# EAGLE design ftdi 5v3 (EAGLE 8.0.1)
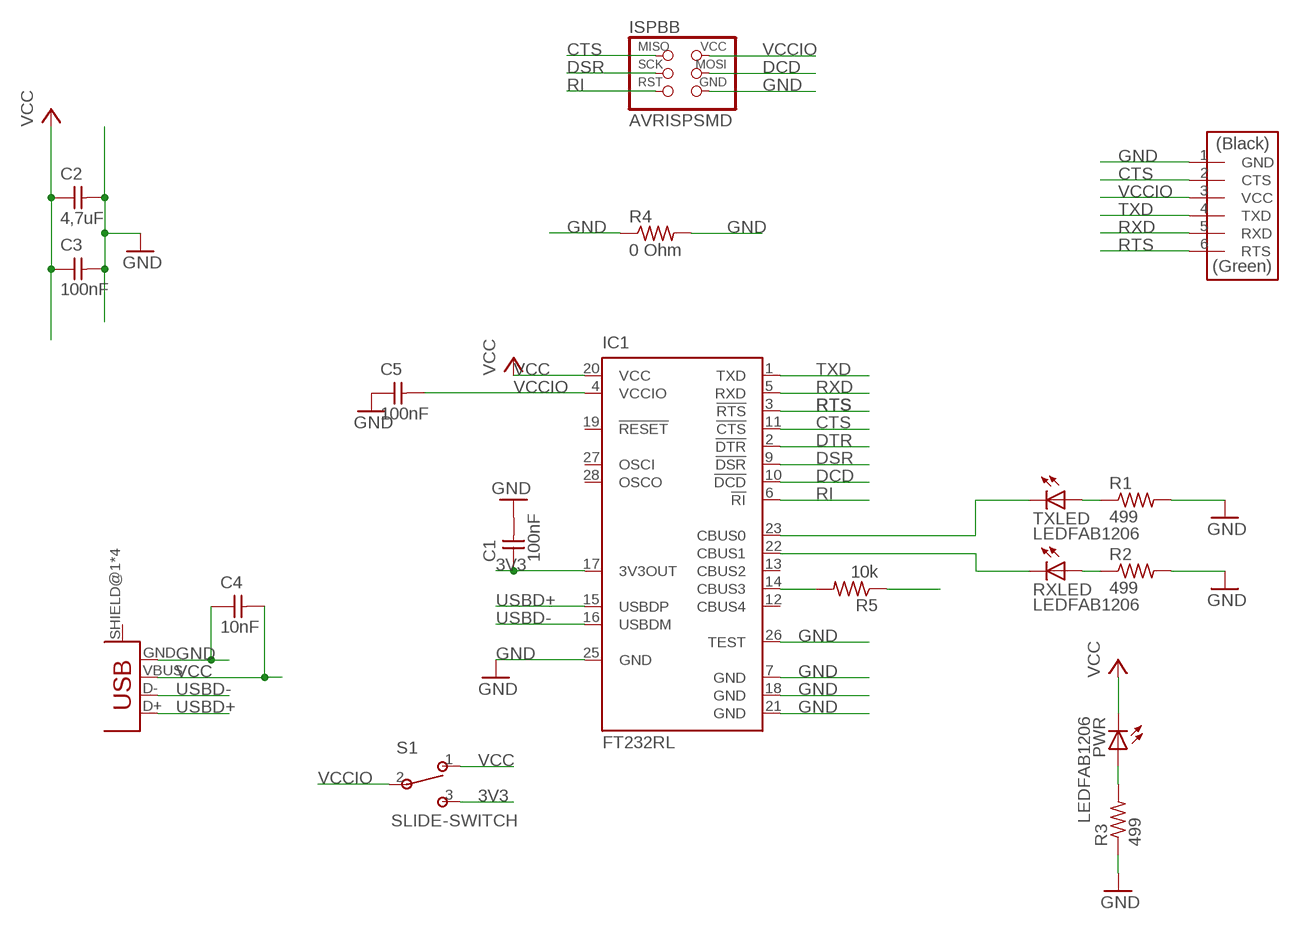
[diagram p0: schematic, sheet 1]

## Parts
C1  100nF  CAP-UNPOLARIZEDFAB  [C1206FAB]
C2  4,7uF  CAP-UNPOLARIZEDFAB  [C1206FAB]
C3  100nF  CAP-UNPOLARIZEDFAB  [C1206FAB]
C4  10nF  CAP-UNPOLARIZEDFAB  [C1206FAB]
C5  100nF  CAP-UNPOLARIZEDFAB  [C1206FAB]
FTDI  FTDI-SMD-HEADER  [1X06SMD]
IC1  FT232RL  [SSOP28]
ISPBB  AVRISPSMD  [2X03SMD]
PWR  LEDFAB1206  [LED1206FAB]
R1  499  RES-US1206FAB  [R1206FAB]
R2  499  RES-US1206FAB  [R1206FAB]
R3  499  RES-US1206FAB  [R1206FAB]
R4  0 Ohm  RES-US1206FAB  [R1206FAB]
R5  10k  RES-US1206FAB  [R1206FAB]
RXLED  LEDFAB1206  [LED1206FAB]
S1  SLIDE-SWITCH  [AYZ0102AGRLC]
TXLED  LEDFAB1206  [LED1206FAB]
U$5  USB_MINIB  [USB_MINIB]

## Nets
3V3: C1.1 IC1.17(3V3OUT) S1.3
CTS: FTDI.2(CTS) IC1.11(!CTS) ISPBB.1(MISO)
DCD: IC1.10(!DCD) ISPBB.4(MOSI)
DSR: IC1.9(!DSR) ISPBB.3(SCK)
DTR: IC1.2(!DTR)
GND: C1.2 C2.2 C3.2 C4.1 C5.1 FTDI.1(GND) IC1.7(GND) IC1.18(GND) IC1.21(GND) IC1.25(GND) IC1.26(TEST) ISPBB.6(GND) R1.2 R2.2 R3.1 R4.1 R4.2 U$5.GND
N$1: PWR.1(A) R3.2
N$2: IC1.14(CBUS3) R5.2
N$17: IC1.23(CBUS0) TXLED.2(C)
N$18: IC1.22(CBUS1) RXLED.2(C)
N$20: R2.1 RXLED.1(A)
N$21: R1.1 TXLED.1(A)
RI: IC1.6(!RI) ISPBB.5(RST)
RTS: FTDI.6(RTS) IC1.3(!RTS)
RXD: FTDI.5(RXD) IC1.5(RXD)
TXD: FTDI.4(TXD) IC1.1(TXD)
USBD+: IC1.15(USBDP) U$5.D+
USBD-: IC1.16(USBDM) U$5.D-
VCC: C2.1 C3.1 C4.2 IC1.20(VCC) PWR.2(C) S1.1 U$5.VBUS
VCCIO: C5.2 FTDI.3(VCC) IC1.4(VCCIO) ISPBB.2(VCC) R5.1 S1.2
Unconnected: IC1.12(CBUS4) IC1.13(CBUS2) IC1.19(!RESET) IC1.27(OSCI) IC1.28(OSCO) U$5.SHIELD@1(SHIELD) U$5.SHIELD@2(SHIELD) U$5.SHIELD@3(SHIELD) U$5.SHIELD@4(SHIELD)

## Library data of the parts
C1-C5 = fab:CAP-UNPOLARIZED
FTDI = fab:FTDI-SMD-HEADER
IC1 = ftdichip:FT232R: Source: http://www.ftdichip.com/Documents/DataSheets/DS_FT232R_v104.pdf; MPN: FT232RL; OC_FARNELL: 1146032; OC_NEWARK: 91K9918
ISPBB = fab:AVRISP
PWR RXLED TXLED = fab:LED: LED
R1-R5 = fab:RES-US: Resistor (US Symbol)
S1 = fab:SLIDE-SWITCH: SMD slide-switch AYZ0102AGRLC as found in the fablab inventory. Includes the mounting holes. Made by Zaerc.
U$5 = fab:USB_MINIB

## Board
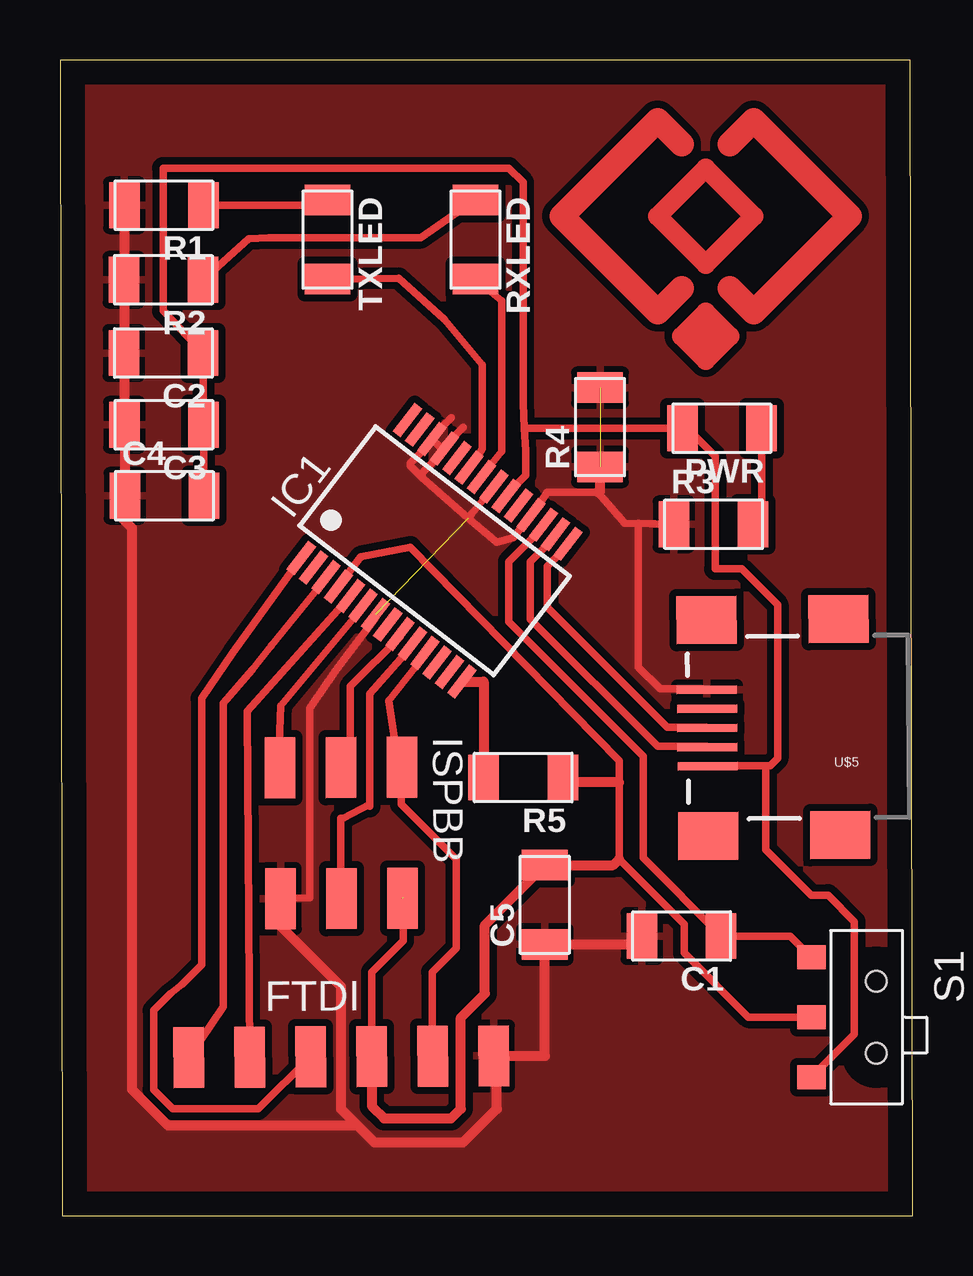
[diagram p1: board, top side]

Size 35.53 x 48.15 mm. Coordinates in mm from the lower left corner, seen from the top.
Outline: 0.1,0 35.53,0 35.43,48.15 0,48.15 0.1,0
Copper layers (1*16): Top 0.035mm / dielectric 1.5mm / Bottom 0.035mm
Design rules "thight *": minimum track width 0.3mm, minimum drill 24mil, track to track 0.3mm, track to pad 0.3mm, pad to pad 8mil, via to via 8mil, smd to smd 0.3mm, copper to edge 40mil, drill to drill 8mil, minimum pad ring 10mil, minimum via ring 8mil, stop-mask expansion 4mil, vias tented up to drill 0mil, thermal gap 10mil

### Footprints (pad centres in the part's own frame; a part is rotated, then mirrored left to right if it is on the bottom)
C1206FAB = smd 1.27 x 1.905: 1 -1.651,0; 2 1.651,0
1X06SMD = smd 2.54 x 1.27: 1 0,6.35; 2 0,3.81; 3 0,1.27; 4 0,-1.27; 5 0,-3.81; 6 0,-6.35
SSOP28 = smd 0.4 x 1.5: 1 -4.225,-3.625; 2 -3.575,-3.625; 3 -2.925,-3.625; 4 -2.275,-3.625; 5 -1.625,-3.625; 6 -0.975,-3.625; 7 -0.325,-3.625; 8 0.325,-3.625; 9 0.975,-3.625; 10 1.625,-3.625; 11 2.275,-3.625; 12 2.925,-3.625; 13 3.575,-3.625; 14 4.225,-3.625; 15 4.225,3.625; 16 3.575,3.625; 17 2.925,3.625; 18 2.275,3.625; 19 1.625,3.625; 20 0.975,3.625; 21 0.325,3.625; 22 -0.325,3.625; 23 -0.975,3.625; 24 -1.625,3.625; 25 -2.275,3.625; 26 -2.925,3.625; 27 -3.575,3.625; 28 -4.225,3.625
2X03SMD = smd 2.54 x 1.27: 1 -2.54,2.54; 2 2.92,2.54; 3 -2.54,0; 4 2.92,0; 5 -2.54,-2.54; 6 2.92,-2.54
LED1206FAB = smd 1.27 x 1.905: 1 -1.651,0; 2 1.651,0
R1206FAB = smd 1.27 x 1.905: 1 -1.651,0; 2 1.651,0
AYZ0102AGRLC = smd 1 x 1.2: 1 2.5,-2.3; 2 0,-2.3; 3 -2.5,-2.3 | hole 0.85: -1.5,0.4; 1.5,0.4
USB_MINIB = smd 2.5 x 0.35: D+ 3.77,0; D- 3.77,0.8; GND 3.77,-1.6; ID 3.77,-0.8; VBUS 3.77,1.6 | smd 2.5 x 2: SHIELD@1 -1.73,-4.5; SHIELD@2 -1.73,4.5; SHIELD@3 3.77,4.5; SHIELD@4 3.77,-4.5

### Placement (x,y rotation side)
C1  25.9,11.65 180 top
C2  4.31,35.94 180 top
C3  4.33,32.95 180 top
C4  4.35,29.99 0 top
C5  20.2,12.95 90 top
FTDI  11.72,6.62 270.3 top
IC1  15.61,27.7 322.4 top
ISPBB  11.72,16.13 270.2 top
PWR  27.58,32.81 180 top
R1  4.33,42.1 180 top
R2  4.31,38.99 180 top
R3  27.23,28.81 0 top
R4  22.5,32.85 90 top
R5  19.3,18.25 180 top
RXLED  17.31,40.67 270 top
S1  33.61,8.27 270 top
TXLED  11.15,40.67 270 top
U$5  30.74,20.35 180.5 top

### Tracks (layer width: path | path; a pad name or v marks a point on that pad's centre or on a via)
3V3
  Top 0.305: IC1.17 20.14,28.69 18.7,27.25 18.7,24.75 24.3,19.15 24.3,14.9 C1.1 30.43,11.65 S1.3
CTS
  Top 0.305: IC1.11 15.2,23.35 13.7,21.45 14.1,18.83 ISPBB.1 14.21,17.13 16.5,14.85 16.5,11.15 15.5,10.15 15.5,6.56 FTDI.2
DCD
  Top 0.305: IC1.10 14.69,23.74 12.9,21.75 12.9,17.15 | 12.9,17.05 12.9,17.15 | 12.9,17.15 11.8,16.55 11.7,16.55 11.7,13.28 ISPBB.4
DSR
  Top 0.305: IC1.9 14.17,24.12 12.1,22.05 12.1,19.09 ISPBB.3
GND  (2 unrouted)
  Top 0.305: IC1.25 15.9,31.96 IC1.26 | U$5.GND 26.79,21.95 25,21.95 24.1,22.85 24.1,28.85 25.56,28.81 R3.1 23.54,28.85 22.4,30.15 20.3,30.15 19.92,29.57 IC1.18 18.89,28.25 18.2,28.05 17,29.05 | IC1.7 13.14,24.89 11.5,22.75 11.1,22.15 10.4,21.15 10.4,13.24 ISPBB.6 | IC1.25 16.02,31.87 15.1,30.95 15.1,30.75 | 17,29.05 17.16,29.25 IC1.21 | 15.1,30.75 17,29.05 | IC1.26 15.5,32.45 16.3,33.25 | IC1.25 16.02,32.07 16.8,32.85 | IC1.26 15.5,32.25 14.6,31.35 14.6,31.25 15.1,30.75
  Top 0.406: 22.4,30.15 22.5,30.15 R4.1 | ISPBB.6 9.19,12.06 11.7,9.55 11.7,4.45 12.4,3.75 | 12.4,3.75 13.1,3.05 16.8,3.05 18.2,4.45 18.2,6.52 FTDI.1 20.2,6.65 C5.1 24.25,11.3 C1.2 | 12.4,3.75 4.5,3.75 3,5.25 3,28.65 2.4,29.25 2.4,29.69 C4.1 2.7,33.05 | 2.7,35.75 2.7,38.95 | 2.7,33.05 2.7,35.75 | 2.7,38.95 2.7,42.08 R1.2 | R2.2 2.7,38.95 | C2.2 2.66,35.79 2.7,35.75 | C3.2 2.68,33.03 2.7,33.05
  pour Top (isolate 0.305): 0.2,0.15 35.3,0.15 35.3,47.95 0.2,47.95
N$1
  Top 0.305: PWR.1 29.23,29.16 R3.2
N$2
  Top 0.406: IC1.14 17.65,22.25 R5.2
N$3
  Top 0.61: 26.9,37.65 26.9,35.65 | 25.9,36.65 27.9,36.65
  Top 0.813: 26.9,37.65 25.9,36.65 26.9,35.65 27.9,36.65 26.9,37.65
N$4
  Top 1.016: 25.9,38.65 24.9,37.65 20.9,41.65 24.9,45.65 25.9,44.65
N$5
  Top 0.813: 26.9,43.65 24.9,41.65 26.9,39.65 28.9,41.65 26.9,43.65
N$6
  Top 1.016: 27.9,44.65 28.9,45.65 32.9,41.65 28.9,37.65 27.9,38.65
N$17
  Top 0.305: IC1.23 17.45,31.7 17.6,31.95 17.6,35.45 16,37.35 14.12,39.05 TXLED.2
N$18
  Top 0.305: IC1.22 17.56,30.81 18.4,31.85 18.4,38.13 RXLED.2
N$20
  Top 0.305: R2.1 7.86,40.71 8.7,40.75 15.04,40.75 RXLED.1
N$21
  Top 0.305: R1.1 10.83,42.1 TXLED.1
RI
  Top 0.305: IC1.6 12.63,25.38 9.2,21.25 9.1,18.66 ISPBB.5
RTS
  Top 0.305: IC1.3 11.08,26.53 8.8,23.75 8,22.75 6.8,21.35 6.8,8.69 FTDI.6
RXD
  Top 0.305: FTDI.5 7.81,21.02 IC1.5
TXD
  Top 0.305: IC1.1 10.05,27.3 10,27.35 7.2,23.45 5.9,21.55 5.9,10.45 5.1,9.65 4.6,9.25 3.9,8.55 3.9,5.25 4.7,4.45 8.25,4.45 FTDI.4
USBD+
  Top 0.305: IC1.15 21.17,27.92 20.3,27.05 20.3,25.35 25.3,20.35 26.94,20.35 U$5.D+
USBD-
  Top 0.305: IC1.16 20.65,28.3 19.6,27.25 19.6,24.85 24.9,19.55 26.94,19.55 U$5.D-
VCC
  Top 0.305: 29.4,18.75 29.6,18.75 29.9,19.05 29.9,25.45 28.4,26.95 27.3,26.95 27.3,31.65 26.14,32.81 PWR.2 19.34,32.81 | 29.4,18.75 27.02,18.75 U$5.VBUS | 29.4,18.75 29.4,15.25 31.3,13.35 32,13.35 33.1,12.25 33.1,7.56 S1.1 | 19.34,32.81 19.3,33.85 19.3,43.05 18.7,43.65 4.3,43.65 4.3,37.7 C2.1 5.96,32.97 C3.1 5.98,30.01 C4.2 | IC1.20 18.59,30.04 19.4,30.85 19.4,31.87 19.34,32.81
VCCIO  (1 unrouted)
  Top 0.305: S1.2 28.68,8.27 26,10.95 26,12.15 23.3,14.85 23.3,18.05 23.3,18.95 14.6,27.85 12.53,27.45 IC1.4 | FTDI.3 12.99,10.14 14.3,11.45 14.3,13.24
  Top 0.406: 23.3,18.05 20.95,18.05 R5.1 | FTDI.3 12.99,4.56 13.5,4.05 16.3,4.05 16.7,4.45 16.7,8.25 17.7,9.25 17.7,12.1 C5.2 23.05,14.6 23.3,14.85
